PROGRAM MAIN
VAR
	ToPC2 AT %Q*:ARRAY[0..127] OF BYTE;	//发布的数据
	fbTON1: TON;
	q1: BOOL;	
	FromPC2 AT %I*:ARRAY[0..127] OF BYTE;	//接收的数据
	fbTON2: TON;
	fbTON3: TON;
	ComError: BOOL;	// 通信错误
END_VAR

fbTON1(IN:=NOT fbTON1.Q , PT:=T#500MS , Q=> , ET=> );
IF fbTON1.Q THEN
	q1:=NOT q1;
END_IF
ToPC2[0].0:=q1;

//心跳检测
fbTON2(IN:=NOT FromPC2[0].0 , PT:=T#1S , Q=> , ET=> );
fbTON3(IN:=FromPC2[0].0 , PT:=T#1S , Q=> , ET=> );
IF fbTON2.Q OR fbTON3.Q THEN
	ComError:=TRUE;
ELSE
	ComError:=FALSE;
END_IF

END_PROGRAM
